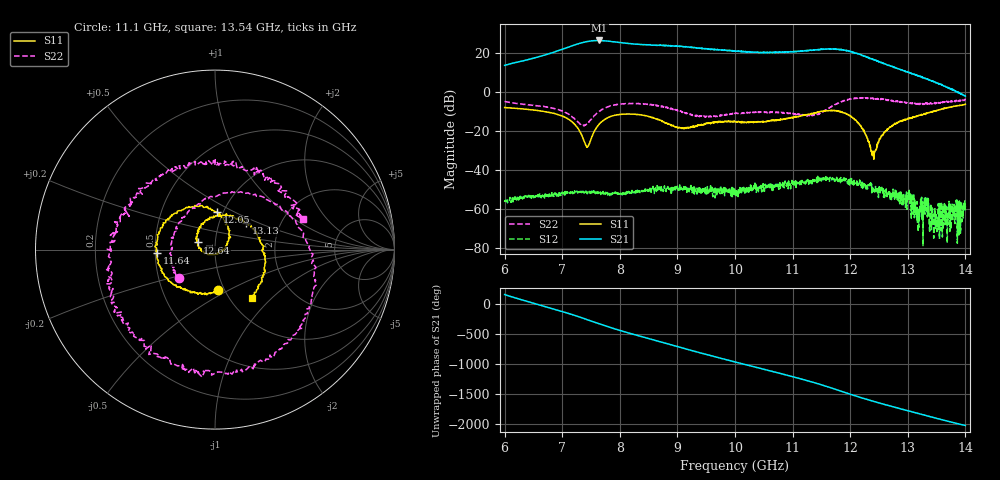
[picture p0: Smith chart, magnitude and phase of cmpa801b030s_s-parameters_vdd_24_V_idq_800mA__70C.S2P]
!Keysight Technologies,E5071C,MY46110325,B.14.03
!Date: Fri Aug 07 15:50:32 2020
!Data & Calibration Information:
!Freq	S11:SOLT2(ON)	S21:SOLT2(ON)	S12:SOLT2(ON)	S22:SOLT2(ON)
!PortZ  Port1:50+j0  Port2:50+j0
!Above PortZ is port z conversion or system Z0 setting when saving the data.
!When reading, reference impedance value at option line is always used.
# Hz S dB R 50
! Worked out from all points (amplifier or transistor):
!   1601 points, 6 GHz to 14 GHz, reference 50 ohm
!   highest |S21| = 26.2 dB at 7.645 GHz (marker M1)
!   |S21| within 3 dB of that: 7.146 GHz to 8.985 GHz (1.839 GHz wide, 22.8 % of centre)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
!   unconditionally stable (mu >= 1): start of sweep to end of sweep
!   at 7.33 GHz: K = 10.73, MAG = 25.1 dB, |S12| = -51.8 dB
!   at 10 GHz: K = 18.03, MAG = 21.3 dB, |S12| = -52.9 dB
!   at 14 GHz: K = 270.19, MAG = 0.9 dB, |S12| = -58.8 dB
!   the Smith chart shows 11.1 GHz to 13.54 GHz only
!   S11 on the Smith chart (normalised r, x): 11.1 GHz: 0.93, -0.44; 11.64 GHz: 0.51, -0.02; 12.05 GHz: 0.94, +0.41; 12.64 GHz: 0.82, +0.07; 13.13 GHz: 1.35, +0.42; 13.54 GHz: 1.26, -0.77
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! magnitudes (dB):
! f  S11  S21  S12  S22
! 6 GHz  -8.2  13.5  -56.6  -5.0
! 6.965 GHz  -12.2  21.3  -52.0  -9.5
! 7.335 GHz  -22.2  25.0  -51.7  -17.1
! 7.445 GHz  -28.2  25.7  -51.4  -15.9
! 7.645 GHz  -16.6  26.2  -52.1  -10.1
! 8.065 GHz  -11.5  25.0  -52.2  -6.3
! 8.67 GHz  -14.4  23.8  -50.1  -7.2
! 9.1 GHz  -18.7  23.0  -50.3  -10.7
! 10 GHz  -15.4  20.8  -52.9  -11.2
! 11.1 GHz  -12.9  20.8  -46.7  -11.8
! 11.34 GHz  -11.4  21.3  -47.4  -12.2
! 11.64 GHz  -9.8  21.9  -46.0  -8.3
! 12.05 GHz  -13.6  20.3  -45.6  -3.5
! 12.39 GHz  -30.5  16.6  -50.6  -3.5
! 12.64 GHz  -19.6  13.7  -53.2  -4.3
! 12.67 GHz  -18.7  13.6  -52.7  -4.2
! 13.13 GHz  -12.8  8.6  -56.8  -6.0
! 13.32 GHz  -11.0  6.6  -56.8  -6.0
! 13.48 GHz  -9.8  4.8  -70.2  -6.0
! 13.54 GHz  -9.4  4.3  -67.4  -5.7
! 13.9 GHz  -7.2  -0.9  -63.8  -4.4
! 14 GHz  -6.5  -2.3  -58.8  -4.2
